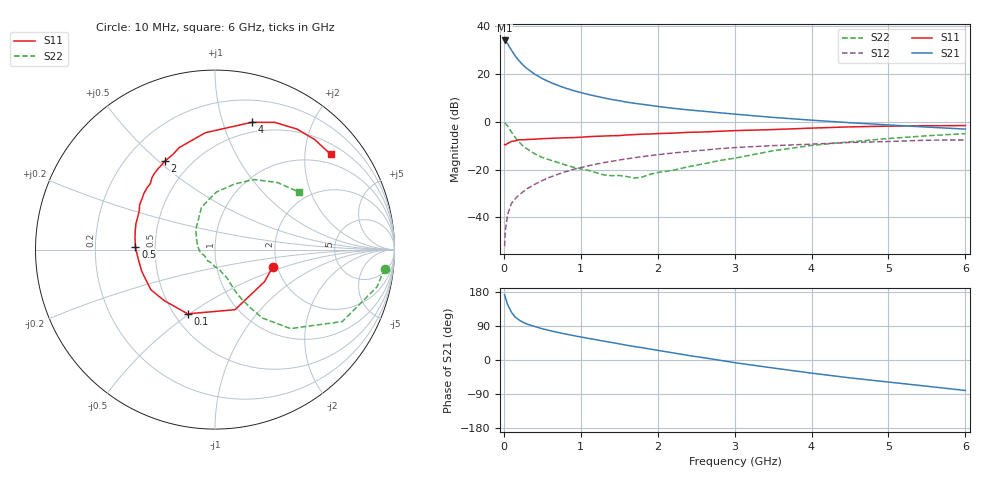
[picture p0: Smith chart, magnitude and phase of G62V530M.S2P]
! SIEMENS Small Signal Semiconductors
! BFG193
! Si NPN RF Bipolar Junction Transistor in SOT223
! VCE = 2.5 V  IC = 30 mA
! Common Emitter S-Parameters:  August  1996
# GHz  S  MA  R  50
!  f  S11  S21  S12  S22
! GHz  MAG  ANG  MAG  ANG  MAG  ANG  MAG  ANG
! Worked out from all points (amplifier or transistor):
!   36 points, 10 MHz to 6 GHz, reference 50 ohm
!   highest |S21| = 34.0 dB at 10 MHz (marker M1)
!   |S21| within 3 dB of that: start of sweep to 79.41 MHz
!   unconditionally stable (mu >= 1): 555.9 MHz to 2.541 GHz
!   at 250 MHz: K = 0.85, MSG = 26.5 dB, |S12| = -29.3 dB
!   at 1.4 GHz: K = 1.05, MAG = 11.6 dB, |S12| = -16.6 dB
!   at 6 GHz: K = 0.91, MSG = 2.3 dB, |S12| = -7.6 dB
!   S11 on the Smith chart (normalised r, x): 10 MHz: 1.89, -0.41; 100 MHz: 0.58, -0.49; 500 MHz: 0.38, +0.02; 2 GHz: 0.36, +0.53; 4 GHz: 0.40, +1.25; 6 GHz: 0.74, +2.60
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0.01  0.3359 -16.5  50.36 171.9  0.0025 89.7  0.951 -6.4
0.02  0.3289 -32.8  49.14 165.1  0.0054 83.1  0.9259 -13.0
0.05  0.3529 -71.6  42.62 145.5  0.0117 70.0  0.8143 -29.5
0.1  0.3888 -113.0  31.46 125.7  0.0198 63.4  0.6086 -46.3
0.15  0.4006 -134.6  23.55 112.8  0.0248 61.8  0.4638 -55.3
0.2  0.4213 -147.8  18.75 105.3  0.0297 62.5  0.377 -58.8
0.25  0.4208 -157.3  15.38 99.4  0.0343 62.6  0.3114 -61.7
0.3  0.4259 -164.0  13.03 95.0  0.0396 64.3  0.2724 -63.5
0.4  0.4324 -174.3  9.962 88.5  0.0491 64.5  0.2144 -65.4
0.5  0.4442 177.8  8.023 82.4  0.059 64.0  0.1795 -66.6
0.6  0.4503 171.7  6.737 77.5  0.0697 63.7  0.1588 -68.6
0.8  0.4638 161.5  5.074 68.6  0.0899 61.1  0.125 -75.0
1.1  0.4891 149.2  3.727 57.1  0.1202 56.3  0.0963 -90.0
1.6  0.5315 131.5  2.577 38.9  0.1683 46.1  0.0714 -132.7
2  0.567 119.4  2.1 25.5  0.205 37.2  0.0869 -175.9
2.2  0.5791 114.0  1.915 18.8  0.2226 32.6  0.0966 170.4
3  0.6536 94.6  1.448 -7.0  0.2888 14.3  0.173 124.9
3.5  0.6882 82.8  1.237 -21.1  0.3176 1.4  0.2481 107.7
4  0.7385 73.8  1.082 -34.7  0.3407 -8.3  0.3204 88.7
4.5  0.7833 64.8  0.957 -47.2  0.3699 -18.4  0.3813 73.4
5.5  0.8275 47.8  0.776 -69.2  0.4125 -41.5  0.5099 47.2
6  0.8346 39.5  0.704 -80.4  0.4172 -54.8  0.5665 34.6
